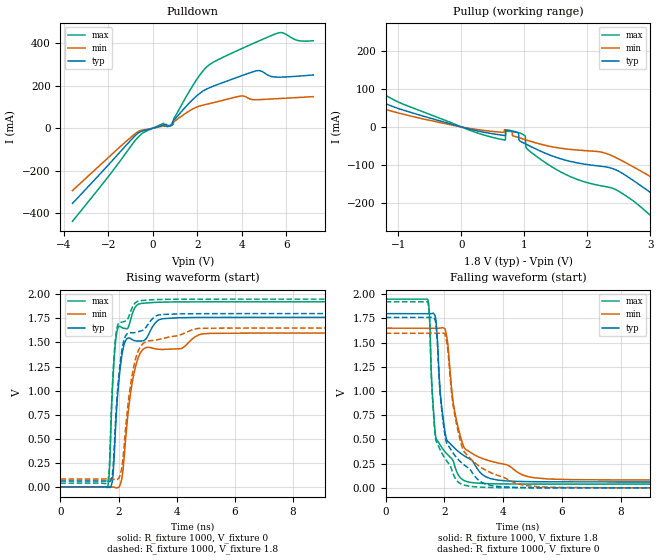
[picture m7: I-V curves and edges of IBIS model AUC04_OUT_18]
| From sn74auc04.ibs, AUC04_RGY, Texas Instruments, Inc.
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[Model]   AUC04_OUT_18
Model_type  Output
Vref =   0
Rref =   1000
Cref =   30p
Vmeas =   0.9
| variable   typ   min   max
C_comp   3.5pF   NA   NA
| C_pullup   8.40pF   1.40pF   22.32pF
| C_pulldown   6.69pF   0.86pF   15.74pF
[Temperature Range]   40   100   -40
| Ambient temperature   25   85   -40
[Voltage range]   1.8   1.65   1.95
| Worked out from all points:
|   slope of the pulldown table from 0 to 0.27 V, typ, clamps not added: 34.3 ohm
|   slope of the pullup table from 0 to 0.27 V, typ, clamps not added: 24.6 ohm
|   rising waveform, R_fixture 1000, V_fixture 0: 20-80 % time 284ps typ, 414ps min, 194ps max; typ from 0 V to 1.76 V
|   falling waveform, R_fixture 1000, V_fixture 1.8: 20-80 % time 576ps typ, 581ps min, 384ps max; typ from 1.8 V to 0.061 V
|   rising waveform, R_fixture 1000, V_fixture 1.8: 20-80 % time 282ps typ, 410ps min, 193ps max; typ from 0.061 V to 1.8 V
|   falling waveform, R_fixture 1000, V_fixture 0: 20-80 % time 539ps typ, 673ps min, 352ps max; typ from 1.76 V to 0 V
[Pulldown]
| AUC04_OUT_18
|   Voltage   I(typ)   I(min)   I(max)
-3.6V     -353mA     -292.5mA   -437.1mA
-555mV    -16.57mA   -11mA      -31.66mA
495mV     15.16mA    11.03mA    23.58mA
820mV     12.51mA    12.73mA    14.89mA
925mV     35.08mA    28.52mA    18.81mA
950mV     37.73mA    30.39mA    46.5mA
1.675V    122.4mA    83.44mA    179.3mA
2.51V     188.6mA    114.9mA    296mA
3.98V     246.3mA    151.7mA    373.5mA
4.685V    270.2mA    134mA      406.4mA
5.665V    240.1mA    139.5mA    448.4mA
7.2V      250.2mA    148.3mA    411mA
[Pullup]
| AUC04_OUT_18
|   Voltage   I(typ)   I(min)   I(max)
-3.6V     279.3mA    234.4mA    328.1mA
-2.85V    204.9mA    166.3mA    251mA
-1.38V    73.83mA    55.65mA    100.5mA
375mV     -14.45mA   -9.607mA   -22.05mA
940mV     -38.19mA   -29.59mA   -16.84mA
1.015V    -44.32mA   -33.6mA    -24.07mA
1.045V    -46.82mA   -35.18mA   -57.98mA
1.425V    -75.29mA   -51.77mA   -103.9mA
2.46V     -113.6mA   -81.44mA   -165.9mA
3.345V    -213mA     -163.7mA   -282.3mA
4.39V     -335.7mA   -266.5mA   -428.1mA
7.2V      -660.5mA   -545mA     -809.4mA
[Ramp]
| AUC04_OUT_18
| variable   typ   min   max
dV/dt_r   1.06/2.87E-10   0.96/4.17E-10   1.16/2.00E-10
dV/dt_f   1.05/5.76E-10   0.94/5.83E-10   1.15/3.85E-10
R_load = 1000
[Rising Waveform]
| AUC04_OUT_18
R_fixture =   1000
C_fixture =   0
L_fixture =   0
V_fixture =   0
V_fixture_min = 0
V_fixture_max = 0
|   Time   V(typ)   V(min)   V(max)
0s        10.21nV    35.63nV    1.217nV
1.625ns   -3.358mV   952.8uV    -3.521mV
1.685ns   -5.635mV   904.5uV    160.1mV
1.795ns   70.51mV    -1.125mV   1.048V
1.935ns   809.9mV    -10.3mV    1.595V
2.205ns   1.49V      343.1mV    1.646V
2.415ns   1.54V      973.2mV    1.733V
2.705ns   1.514V     1.362V     1.9V
3.94ns    1.755V     1.433V     1.921V
22.5ns    1.761V     1.597V     1.922V
[Falling Waveform]
| AUC04_OUT_18
R_fixture =   1000
C_fixture =   0
L_fixture =   0
V_fixture =   1.8
V_fixture_min = 1.65
V_fixture_max = 1.95
|   Time   V(typ)   V(min)   V(max)
0s        1.8V       1.65V      1.95V
1.43ns    1.8V       1.65V      1.95V
1.585ns   1.802V     1.649V     991.3mV
1.71ns    1.727V     1.649V     516.3mV
1.865ns   961.6mV    1.651V     437.6mV
2.055ns   522.5mV    1.6V       360.8mV
2.345ns   410.5mV    795.1mV    231.8mV
2.78ns    311.9mV    387.3mV    63.62mV
5.545ns   62.51mV    91.45mV    39.03mV
22.5ns    61.11mV    81.04mV    38.71mV
[Rising Waveform]
| AUC04_OUT_18
R_fixture =   1000
C_fixture =   0
L_fixture =   0
V_fixture =   1.8
V_fixture_min = 1.65
V_fixture_max = 1.95
|   Time   V(typ)   V(min)   V(max)
0s        61.05mV    81.01mV    38.68mV
1.625ns   58.06mV    81.82mV    36.77mV
1.685ns   57.26mV    81.76mV    209.9mV
1.795ns   149.2mV    79.99mV    1.084V
1.935ns   873.9mV    74.4mV     1.631V
2.19ns    1.525V     409.1mV    1.717V
2.41ns    1.601V     1.048V     1.816V
2.69ns    1.613V     1.42V      1.931V
4.86ns    1.799V     1.647V     1.95V
22.5ns    1.8V       1.65V      1.95V
[Falling Waveform]
| AUC04_OUT_18
R_fixture =   1000
C_fixture =   0
L_fixture =   0
V_fixture =   0
V_fixture_min = 0
V_fixture_max = 0
|   Time   V(typ)   V(min)   V(max)
0s        1.761V     1.597V     1.922V
1.43ns    1.761V     1.597V     1.921V
1.485ns   1.761V     1.597V     1.787V
1.705ns   1.698V     1.597V     497.4mV
1.86ns    953.3mV    1.599V     389.8mV
2.04ns    504.7mV    1.563V     294.7mV
2.33ns    345.1mV    787.3mV    121.2mV
2.685ns   233mV      368.4mV    26.97mV
5.18ns    1.893mV    12.2mV     435.5uV
22.5ns    59.82uV    23.71uV    26.38uV
